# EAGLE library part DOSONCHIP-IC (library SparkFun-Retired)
DOSonCHIP IC This is the tested schematic and footprint for the DOSonCHIP FAT16 FAT32 IC. Spark Fun Electronics SKU : COM-07956. QFN package also tested/proven.
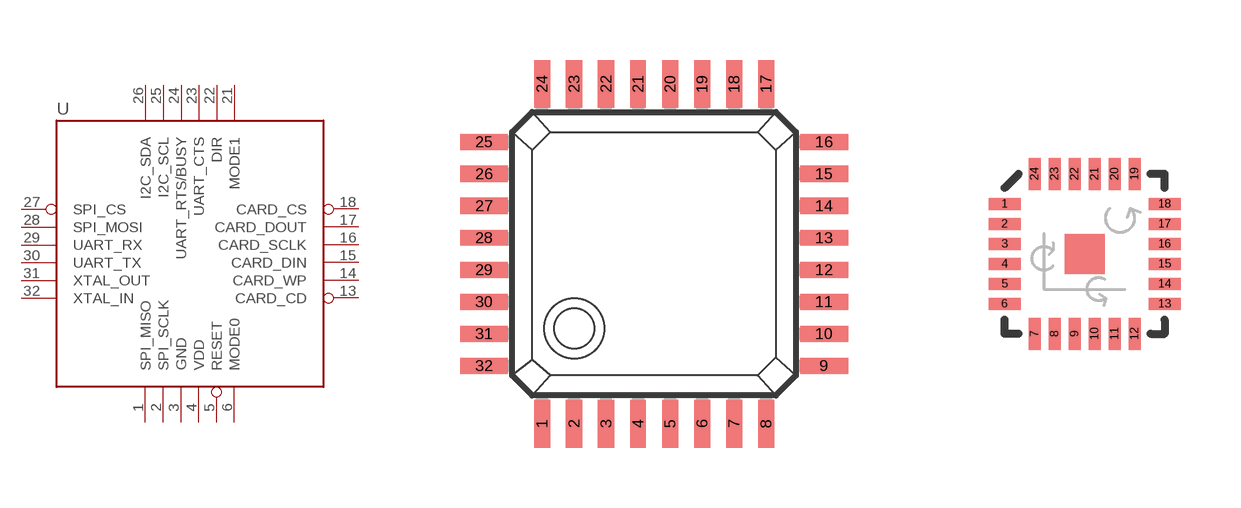
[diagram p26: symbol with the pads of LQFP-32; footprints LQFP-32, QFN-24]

Designator prefix -

## DOSONCHIP-ICLQFP  [LQFP-32]
1  SPI_MISO  out
2  SPI_SCLK  in
3  GND  in
4  VDD  in
5  RESET  in
6  MODE0  in
13  CARD_CD  in
14  CARD_WP  in
15  CARD_DIN
16  CARD_SCLK  out
17  CARD_DOUT  out
18  CARD_CS  in
21  MODE1  in
22  DIR  in
23  UART_CTS  in
24  UART_RTS/BUSY  out
25  I2C_SCL
26  I2C_SDA
27  SPI_CS  in
28  SPI_MOSI  in
29  UART_RX  in
30  UART_TX  out
31  XTAL_OUT  out
32  XTAL_IN  in

## DOSONCHIP-ICQFN  [QFN-24]
1  SPI_MISO  out
2  SPI_SCLK  in
3  GND  in
4  VDD  in
5  RESET  in
6  MODE0  in
7  CARD_CD  in
8  CARD_WP  in
9  CARD_DIN
10  CARD_SCLK  out
11  CARD_DOUT  out
12  CARD_CS  in
13  MODE1  in
14  DIR  in
15  UART_CTS  in
16  UART_RTS/BUSY  out
17  I2C_SCL
18  I2C_SDA
19  SPI_CS  in
20  SPI_MOSI  in
21  UART_RX  in
22  UART_TX  out
23  XTAL_OUT  out
24  XTAL_IN  in

## DOSONCHIP-ICQFN_ALT1  [QFN-24_ALT1.PAC]
Pads as for QFN-24

## Footprint LQFP-32 (pad centres in mm)
Quad Flat Package 32 LD LQFP Source: ds232b12.pdf http://www.ftdichip.com
smd 0.4 x 1.2: 1 -2.8,-4.25; 2 -2,-4.25; 3 -1.2,-4.25; 4 -0.4,-4.25; 5 0.4,-4.25; 6 1.2,-4.25; 7 2,-4.25; 8 2.8,-4.25; 17 2.8,4.25; 18 2,4.25; 19 1.2,4.25; 20 0.4,4.25; 21 -0.4,4.25; 22 -1.2,4.25; 23 -2,4.25; 24 -2.8,4.25
smd 1.2 x 0.4: 9 4.25,-2.8; 10 4.25,-2; 11 4.25,-1.2; 12 4.25,-0.4; 13 4.25,0.4; 14 4.25,1.2; 15 4.25,2; 16 4.25,2.8; 25 -4.25,2.8; 26 -4.25,2; 27 -4.25,1.2; 28 -4.25,0.4; 29 -4.25,-0.4; 30 -4.25,-1.2; 31 -4.25,-2; 32 -4.25,-2.8

## Footprint QFN-24 (pad centres in mm)
smd 0.8 x 0.3: 1 -2,1.25; 2 -2,0.75; 3 -2,0.25; 4 -2,-0.25; 5 -2,-0.75; 6 -2,-1.25; 13 2,-1.25; 14 2,-0.75; 15 2,-0.25; 16 2,0.25; 17 2,0.75; 18 2,1.25
smd 0.3 x 0.8: 7 -1.25,-2; 8 -0.75,-2; 9 -0.25,-2; 10 0.25,-2; 11 0.75,-2; 12 1.25,-2; 19 1.25,2; 20 0.75,2; 21 0.25,2; 22 -0.25,2; 23 -0.75,2; 24 -1.25,2

## Footprint QFN-24_ALT1.PAC (pad centres in mm)
smd 0.851 x 0.3: 1 -2.025,1.25; 2 -2.025,0.75; 3 -2.025,0.25; 4 -2.025,-0.25; 5 -2.025,-0.75; 6 -2.025,-1.25; 13 2.025,-1.25; 14 2.025,-0.75; 15 2.025,-0.25; 16 2.025,0.25; 17 2.025,0.75; 18 2.025,1.25
smd 0.3 x 0.851: 7 -1.25,-2.025; 8 -0.75,-2.025; 9 -0.25,-2.025; 10 0.25,-2.025; 11 0.75,-2.025; 12 1.25,-2.025; 19 1.25,2.025; 20 0.75,2.025; 21 0.25,2.025; 22 -0.25,2.025; 23 -0.75,2.025; 24 -1.25,2.025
